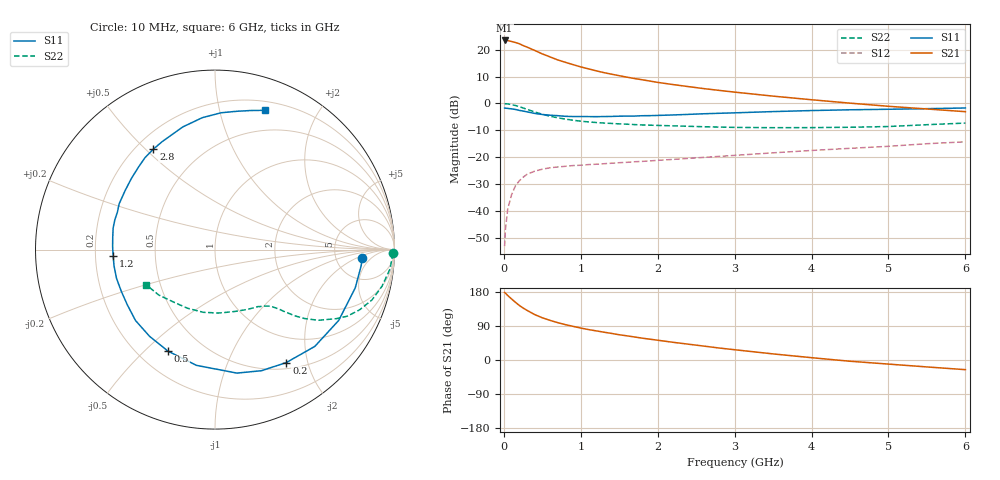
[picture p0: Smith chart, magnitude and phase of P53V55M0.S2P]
! SIEMENS Small Signal Semiconductors
! BFP183
! Si NPN RF Bipolar Junction Transistor in SOT143
! VCE = 3.5 V  IC = 5 mA
! Common Emitter S-Parameters:  March  1996
# GHz  S  MA  R  50
!  f  S11  S21  S12  S22
! GHz  MAG  ANG  MAG  ANG  MAG  ANG  MAG  ANG
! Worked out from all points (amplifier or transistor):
!   36 points, 10 MHz to 6 GHz, reference 50 ohm
!   highest |S21| = 23.5 dB at 10 MHz (marker M1)
!   |S21| within 3 dB of that: start of sweep to 343.5 MHz
!   unconditionally stable (mu >= 1): 1.588 GHz to 5.64 GHz
!   at 250 MHz: K = 0.21, MSG = 24.5 dB, |S12| = -27.5 dB
!   at 1.4 GHz: K = 0.93, MSG = 16.6 dB, |S12| = -22.2 dB
!   at 6 GHz: K = 0.94, MSG = 5.6 dB, |S12| = -14.3 dB
!   lowest NFmin = 1.15 dB at 450 MHz
!   S11 on the Smith chart (normalised r, x): 10 MHz: 9.45, -2.57; 200 MHz: 0.59, -1.66; 500 MHz: 0.32, -0.59; 1.2 GHz: 0.28, -0.03; 2.8 GHz: 0.27, +0.53; 6 GHz: 0.29, +1.38
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0.01  0.8208 -3.1  14.93 178.2  0.0022 85.1  0.9936 -1.2
0.02  0.8195 -6.2  14.87 176.6  0.0044 88.3  0.9885 -2.5
0.05  0.81 -15.3  14.86 170.3  0.0107 83.9  0.9812 -6.3
0.1  0.7942 -29.8  14.29 161.1  0.0199 73.8  0.9526 -12.4
0.15  0.7747 -44.1  13.68 152.4  0.0291 67.2  0.9183 -17.8
0.2  0.7443 -57.7  12.99 144.2  0.0361 62.2  0.8728 -22.6
0.25  0.7228 -69.0  12.02 137.2  0.0423 56.4  0.8255 -26.7
0.3  0.6989 -79.9  11.25 131.2  0.0478 52.1  0.7786 -29.6
0.4  0.6532 -99.1  9.745 119.9  0.0548 45.2  0.697 -34.4
0.5  0.6234 -114.8  8.392 111.4  0.0597 40.3  0.6295 -37.6
0.6  0.6052 -127.1  7.378 104.6  0.0635 36.7  0.5793 -39.6
0.7  0.5934 -138.3  6.485 98.6  0.0657 34.6  0.5413 -40.9
0.9  0.5714 -156.0  5.291 88.8  0.0698 31.7  0.4872 -42.9
1.1  0.5699 -170.7  4.417 80.3  0.0728 30.7  0.4533 -44.8
1.2  0.5685 -176.4  4.061 76.9  0.0739 30.0  0.4422 -45.7
1.7  0.5829 158.6  2.914 60.7  0.0822 30.4  0.4046 -51.7
2.2  0.6114 139.7  2.251 46.7  0.0909 31.2  0.3833 -59.2
2.8  0.6569 121.5  1.753 31.6  0.1034 31.4  0.3635 -70.9
3.5  0.7067 104.7  1.371 16.1  0.1205 30.5  0.354 -87.0
4.5  0.7633 87.4  1.015 -3.3  0.1462 26.7  0.3607 -115.1
5.5  0.8004 75.5  0.79 -18.3  0.1782 22.0  0.4027 -141.1
6  0.8247 70.2  0.704 -25.5  0.1933 18.0  0.4317 -153.2
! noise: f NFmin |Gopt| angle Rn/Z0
0.45  1.15  0.25  40  0.26
0.9  1.2  0.25  93  0.22
1.8  1.95  0.32  170  0.13
